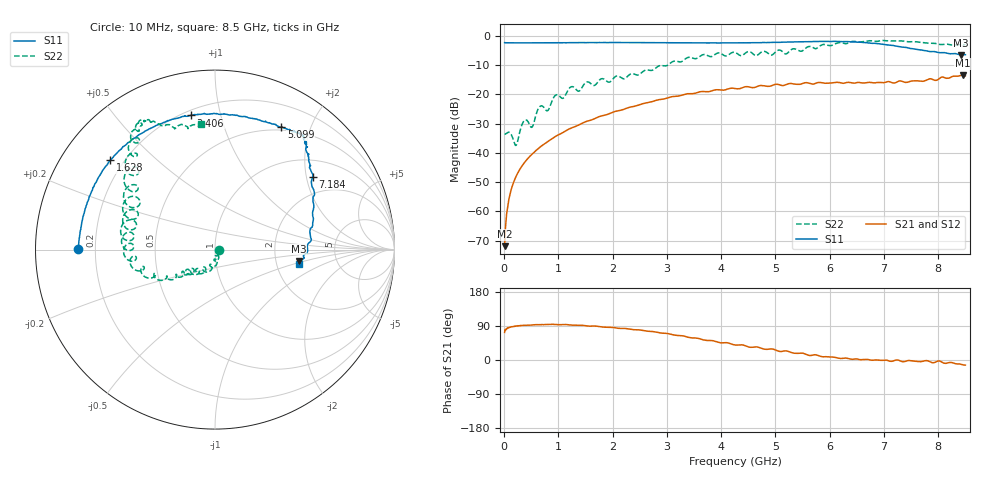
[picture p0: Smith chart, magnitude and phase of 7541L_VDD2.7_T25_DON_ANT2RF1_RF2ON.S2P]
!Agilent Technologies,E5071C,MY46417908,A.11.23
!Date: Wed Dec 09 17:17:32 2020
!Data & Calibration Information:
!Freq	S11:SOLT2(ON)	S21:SOLT2(ON)	S12:SOLT2(ON)	S22:SOLT2(ON)
!PortZ  Port1:50+j0  Port2:50+j0
!Above PortZ is port z conversion or system Z0 setting when saving the data.
!When reading, reference impedance value at option line is always used.
# Hz S dB R 50
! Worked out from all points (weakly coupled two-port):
!   1601 points, 10 MHz to 8.5 GHz, reference 50 ohm
!   highest |S21| = -13.48 dB at 8.447 GHz (marker M1); lowest = -71.9 dB at 10 MHz (marker M2)
!   lowest |S11| = -6.5 dB at 8.415 GHz (marker M3), VSWR 2.78, Z = 135 - j22.1 ohm
!   |S11| at or under -10 dB: nowhere
!   |S22| runs from -37.5 to -1.6 dB; largest |S21 - S12| = 0.0027
!   S11 on the Smith chart (normalised r, x): 10 MHz: 0.13, +0.00; 1.628 GHz: 0.15, +0.36; 3.406 GHz: 0.23, +0.81; 5.099 GHz: 0.46, +1.58; 7.184 GHz: 1.44, +2.18; 8.5 GHz: 2.69, -0.54
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1e7  -2.33 179.6  -71.91 72.7  -72.78 79.1  -33.58 -4.9
6.836875e7  -2.38 178.0  -58.13 84.3  -58.05 83.8  -33.01 -27.8
1.214312e8  -2.39 176.5  -53.15 86.9  -53.25 87.4  -33.41 -49.2
2.2225e8  -2.41 173.6  -48.03 89.6  -47.99 89.7  -37.41 -46.5
3.336812e8  -2.42 170.7  -44.39 91.2  -44.40 91.3  -30.21 -50.0
5.140938e8  -2.41 166.1  -40.48 92.5  -40.48 92.4  -31.19 -74.9
6.520562e8  -2.41 162.5  -38.18 93.4  -38.20 93.4  -24.32 -77.2
8.059375e8  -2.41 158.7  -36.14 93.9  -36.15 94.1  -25.54 -87.2
9.545125e8  -2.39 155.0  -34.32 93.6  -34.33 93.7  -20.23 -96.3
1.426769e9  -2.32 144.0  -29.99 91.8  -30.00 91.8  -17.97 -114.4
1.628406e9  -2.30 139.6  -28.64 89.5  -28.64 89.5  -16.83 -133.3
2.843538e9  -2.34 112.4  -21.86 72.4  -21.87 72.4  -10.38 -146.5
3.406e9  -2.39 100.2  -19.78 59.4  -19.79 59.4  -7.34 -162.3
4.255e9  -2.40 80.6  -18.02 39.7  -18.02 39.6  -5.69 172.0
5.098694e9  -2.20 61.6  -16.89 22.3  -16.85 22.2  -4.99 149.0
5.236656e9  -2.15 60.0  -16.41 22.7  -16.40 22.8  -5.65 153.2
5.671769e9  -1.99 54.7  -16.49 12.3  -16.43 12.2  -3.80 134.4
7.088538e9  -3.16 40.2  -15.64 -2.3  -15.70 -2.3  -1.76 118.9
7.18405e9  -3.36 36.7  -16.14 -1.7  -16.16 -1.5  -1.75 118.9
8.4151e9  -6.54 -7.8  -13.55 -11.0  -13.62 -11.1  -3.04 99.0
8.446938e9  -6.50 -8.5  -13.48 -12.3  -13.56 -12.5  -3.04 98.1
8.5e9  -6.45 -9.4  -13.64 -13.5  -13.73 -13.3  -3.03 96.4
